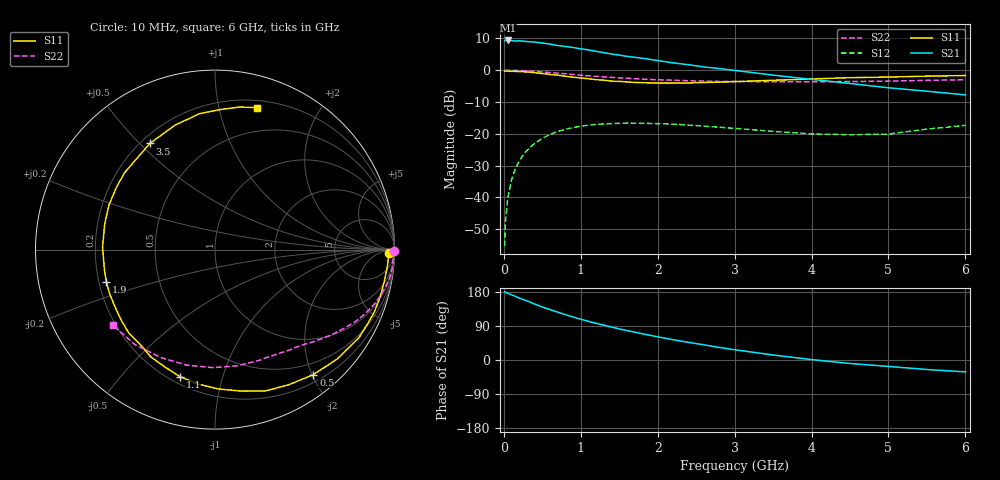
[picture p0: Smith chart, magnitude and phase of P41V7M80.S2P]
! SIEMENS Small Signal Semiconductors
! BFP182
! Si NPN RF Bipolar Junction Transistor in SOT143
! VCE = 1.75 V  IC = 0.8 mA
! Common Emitter S-Parameters:  March  1996
# GHz  S  MA  R  50
!  f  S11  S21  S12  S22
! GHz  MAG  ANG  MAG  ANG  MAG  ANG  MAG  ANG
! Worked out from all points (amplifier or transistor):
!   36 points, 10 MHz to 6 GHz, reference 50 ohm
!   highest |S21| = 9.4 dB at 50 MHz (marker M1)
!   |S21| within 3 dB of that: start of sweep to 1.105 GHz
!   unconditionally stable (mu >= 1): 2.713 GHz to end of sweep
!   at 250 MHz: K = 0.10, MSG = 18.0 dB, |S12| = -26.8 dB
!   at 1.4 GHz: K = 0.53, MSG = 11.0 dB, |S12| = -16.8 dB
!   at 6 GHz: K = 1.10, MAG = 2.8 dB, |S12| = -17.4 dB
!   S11 on the Smith chart (normalised r, x): 10 MHz: 50, -29; 500 MHz: 0.31, -2.02; 1.1 GHz: 0.24, -0.73; 1.9 GHz: 0.23, -0.14; 3.5 GHz: 0.23, +0.54; 6 GHz: 0.26, +1.31
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0.01  0.9703 -1.0  2.925 179.6  0.0017 88.5  0.9987 -0.3
0.02  0.9671 -2.1  2.907 179.0  0.004 87.5  0.9935 -0.7
0.05  0.9654 -5.4  2.94 176.0  0.0096 88.7  0.997 -1.9
0.1  0.9595 -10.6  2.91 171.9  0.0188 81.6  0.993 -4.0
0.2  0.9536 -21.4  2.911 163.5  0.0372 76.5  0.9883 -7.9
0.4  0.9143 -41.7  2.778 147.5  0.0706 64.0  0.9594 -15.2
0.5  0.8865 -51.8  2.676 139.8  0.0847 57.5  0.9388 -18.7
0.6  0.8577 -61.4  2.578 133.0  0.0976 51.8  0.9181 -21.9
0.8  0.8027 -79.2  2.364 119.6  0.1172 41.6  0.8771 -27.4
0.9  0.7772 -88.5  2.278 113.4  0.1251 37.1  0.8551 -29.8
1.1  0.7338 -105.5  2.087 101.9  0.1362 28.7  0.8171 -34.4
1.3  0.6964 -121.0  1.887 91.9  0.1428 21.4  0.785 -38.4
1.5  0.6682 -136.0  1.731 82.1  0.1458 15.2  0.7578 -42.0
1.9  0.6316 -163.4  1.481 65.2  0.1452 5.2  0.7156 -48.8
2.2  0.6266 178.6  1.303 53.5  0.1415 -0.6  0.6962 -53.6
2.8  0.6498 147.7  1.061 33.2  0.1267 -7.9  0.6662 -64.4
3.5  0.694 121.5  0.836 13.2  0.109 -10.1  0.659 -79.1
4  0.7282 107.8  0.718 1.1  0.0993 -5.7  0.6577 -91.0
4.5  0.7625 96.4  0.618 -9.2  0.0966 0.2  0.6631 -103.9
5  0.7809 87.8  0.529 -17.0  0.0989 10.1  0.6735 -116.9
5.5  0.8061 80.2  0.467 -25.1  0.1183 13.3  0.6926 -130.4
6  0.8252 73.4  0.409 -31.4  0.1355 13.1  0.7073 -143.3
